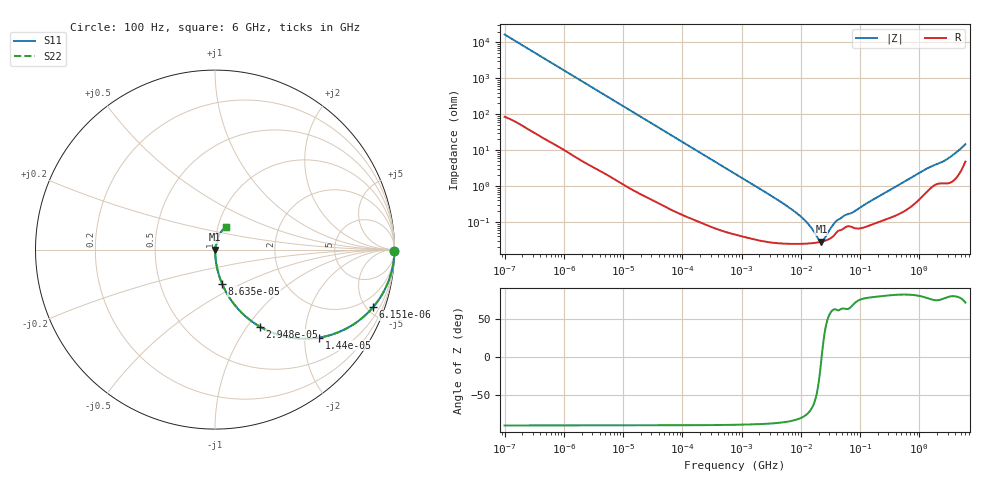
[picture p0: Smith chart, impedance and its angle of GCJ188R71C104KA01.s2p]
!Murata Part Number: GCJ188R71C104KA01
!These Parameters are Measured in Series Mode Connection
!Data Generated on Mar 13, 2026
!  o--ll--o
!Port1  Port2
!  o------o
!Operation Temp=25[degC], DC Bias Voltage=0[V]
!Freq. Start=100[Hz] Stop=6[GHz] 401[Steps]
# Hz S RI R 50
!Freq.(Hz) S11(Real) S11(Imag) S21(Real) S21(Imag) S12(Real) S12(Imag) S22(Real) S22(Imag)
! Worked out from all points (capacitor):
!   401 points, 100 Hz to 6 GHz, reference 50 ohm
!   read as one part in series: C = 95.7 nF near 109 Hz
!   lowest |Z| = 28.5 mohm at 22.26 MHz (marker M1)
!   series resonance near 22.49 MHz, so ESL is about 520 pH
!   S11 on the Smith chart (normalised r, x): 100 Hz: open; 6.151 kHz: 1.04, -5.48; 14.4 kHz: 1.02, -2.35; 29.48 kHz: 1.01, -1.15; 86.35 kHz: 1.00, -0.40; 6 GHz: 1.10, +0.28
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100  0.9999 -0.00603  6.71e-05 0.00603  6.71e-05 0.00603  0.9999 -0.00603
627  0.9984 -0.0374  0.00163 0.0374  0.00163 0.0374  0.9984 -0.0374
2008  0.9852 -0.1177  0.0148 0.1177  0.0148 0.1177  0.9852 -0.1177
6151  0.881 -0.3205  0.119 0.3205  0.119 0.3205  0.881 -0.3205
14402  0.5796 -0.4903  0.4204 0.4903  0.4204 0.4903  0.5796 -0.4903
29482  0.2506 -0.4297  0.7494 0.4297  0.7494 0.4297  0.2506 -0.4297
40335  0.1528 -0.3559  0.8472 0.3559  0.8472 0.3559  0.1528 -0.3559
86348  0.0391 -0.1895  0.9609 0.1895  0.9609 0.1895  0.0391 -0.1895
221108  0.00688 -0.0769  0.9931 0.0769  0.9931 0.0769  0.00688 -0.0769
774597  0.000946 -0.0222  0.9991 0.0222  0.9991 0.0222  0.000946 -0.0222
6644369  0.000254 -0.0024  0.9997 0.0024  0.9997 0.0024  0.000254 -0.0024
1.087309e7  0.000251 -0.00123  0.9997 0.00123  0.9997 0.00123  0.000251 -0.00123
1.555665e7  0.00026 -0.000589  0.9997 0.000589  0.9997 0.000589  0.00026 -0.000589
2.035112e7  0.000276 -0.000157  0.9997 0.000157  0.9997 0.000157  0.000276 -0.000157
2.225763e7  0.000285 -1.61e-05  0.9997 1.61e-05  0.9997 1.61e-05  0.000285 -1.61e-05
2.434276e7  0.000296 0.000125  0.9997 -0.000125  0.9997 -0.000125  0.000296 0.000125
3.482834e7  0.000399 0.000727  0.9996 -0.000727  0.9996 -0.000727  0.000399 0.000727
4.165952e7  0.000556 0.000994  0.9994 -0.000994  0.9994 -0.000994  0.000556 0.000994
3.124326e8  0.00135 0.00754  0.9987 -0.00754  0.9987 -0.00754  0.00135 0.00754
1.251881e9  0.00695 0.028  0.9931 -0.028  0.9931 -0.028  0.00695 0.028
2.802721e9  0.0144 0.0511  0.9856 -0.0511  0.9856 -0.0511  0.0144 0.0511
6e9  0.0626 0.1243  0.9374 -0.1243  0.9374 -0.1243  0.0626 0.1243
